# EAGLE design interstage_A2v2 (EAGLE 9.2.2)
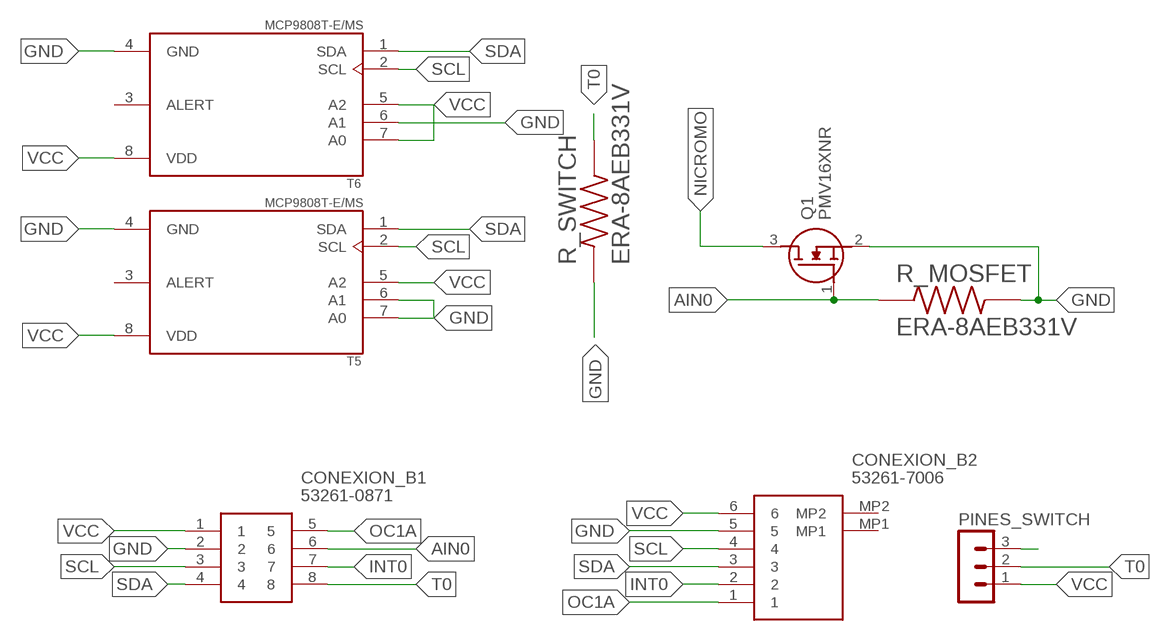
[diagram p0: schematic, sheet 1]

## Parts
CONEXION_B1  53261-0871  [53261-0871]
CONEXION_B2  53261-7006  [532617006]
PINES_SWITCH  MA03-1  [MA03-1]
Q1  PMV16XNR  [SOT95P230X110-3N]
R_MOSFET  ERA-8AEB331V  [RESC3216X70N]
R_SWITCH  ERA-8AEB331V  [RESC3216X70N]
T5  MCP9808T-E/MS  [SOP65P490X110-8N]
T6  MCP9808T-E/MS  [SOP65P490X110-8N]

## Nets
AIN0: CONEXION_B1.6 Q1.1(G) R_MOSFET.1
GND: CONEXION_B1.2 CONEXION_B2.5 Q1.2(S) R_MOSFET.2 R_SWITCH.1 T5.4(GND) T5.6(A1) T5.7(A0) T6.4(GND) T6.6(A1)
INT0: CONEXION_B1.7 CONEXION_B2.2
N$7: PINES_SWITCH.3
NICROMO: Q1.3(D)
OC1A: CONEXION_B1.5 CONEXION_B2.1
SCL: CONEXION_B1.3 CONEXION_B2.4 T5.2(SCL) T6.2(SCL)
SDA: CONEXION_B1.4 CONEXION_B2.3 T5.1(SDA) T6.1(SDA)
T0: CONEXION_B1.8 PINES_SWITCH.2 R_SWITCH.2
VCC: CONEXION_B1.1 CONEXION_B2.6 PINES_SWITCH.1 T5.5(A2) T5.8(VDD) T6.5(A2) T6.7(A0) T6.8(VDD)
Unconnected: CONEXION_B2.MP1 CONEXION_B2.MP2 T5.3(ALERT) T6.3(ALERT)

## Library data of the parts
CONEXION_B1 = SamacSys_Parts:53261-0871: Molex PICOBLADE Series, Series Number 53261, 1.25mm Pitch, 8 Way 1 Row Shrouded Right Angle PCB Header, Surface Mount Source: Datasheet; DESCRIPTION: Molex PICOBLADE Series, Series Number 53261, 1.25mm Pitch, 8 Way 1 Row Shrouded Right Angle PCB Header, Surface Mount; HEIGHT: mm; MANUFACTURER_NAME: Molex; MANUFACTURER_PART_NUMBER: 53261-0871; MOUSER_PART_NUMBER: 538-53261-0871; MOUSER_PRICE-STOCK: https://www.mouser.co.uk/ProductDetail/Molex/53261-0871?qs=%252B72YyncTwW%252BggfdCJ7Netw%3D%3D
CONEXION_B2 = SamacSys_Parts:53261-7006: 1.25mm Pitch, PicoBlade PCB Header, Single Row, Right-Angle, Surface Mount, Gold (Au) Plating, Friction Lock, Circuits, Tape and Reel Source: Datasheet; DESCRIPTION: 1.25mm Pitch, PicoBlade PCB Header, Single Row, Right-Angle, Surface Mount, Gold (Au) Plating, Friction Lock, Circuits, Tape and Reel; HEIGHT: 3.6mm; MANUFACTURER_NAME: Molex; MANUFACTURER_PART_NUMBER: 53261-7006; MOUSER_PART_NUMBER: 538-53261-7006; MOUSER_PRICE-STOCK: https://www.mouser.co.uk/ProductDetail/Molex/53261-7006?qs=0lSvoLzn4L%2FSBef0BTU2GA%3D%3D
PINES_SWITCH = con-lstb:MA03-1: PIN HEADER; OC_FARNELL: unknown; OC_NEWARK: unknown
Q1 = SamacSys_Parts:PMV16XNR: Nexperia PMV16XNR N-channel MOSFET, 8.6 A, 20 V PMV16XN, 3-Pin SOT-23 Source: Datasheet; DESCRIPTION: Nexperia PMV16XNR N-channel MOSFET, 8.6 A, 20 V PMV16XN, 3-Pin SOT-23; HEIGHT: 1.1mm; MANUFACTURER_NAME: Nexperia; MANUFACTURER_PART_NUMBER: PMV16XNR; MOUSER_PART_NUMBER: 771-PMV16XNR; MOUSER_PRICE-STOCK: https://www.mouser.com/Search/Refine.aspx?Keyword=771-PMV16XNR
R_MOSFET R_SWITCH = resistor_330_smd:ERA-8AEB331V; DESCRIPTION: 330 Ohms ±0.1% 0.25W, 1/4W Chip Resistor 1206 (3216 Metric) Automotive AEC-Q200 Thin Film; DIGI-KEY_PART_NUMBER: P330BCCT-ND; MF: Panasonic Electronic; MP: ERA-8AEB331V; PACKAGE: 3216 Panasonic Electronic Components
T5 T6 = sensorSPEL:MCP9808T-E/MS: Board Mount Temperature Sensors Silicon temp sensor with I2C interface; DESCRIPTION: Temperature Sensor Digital, Local -40°C ~ 125°C 10 b 8-MSOP; DIGI-KEY_PART_NUMBER: MCP9808T-E/MSCT-ND; MF: Microchip; MP: MCP9808T-E/MS; PACKAGE: MSOP-8 Microchip

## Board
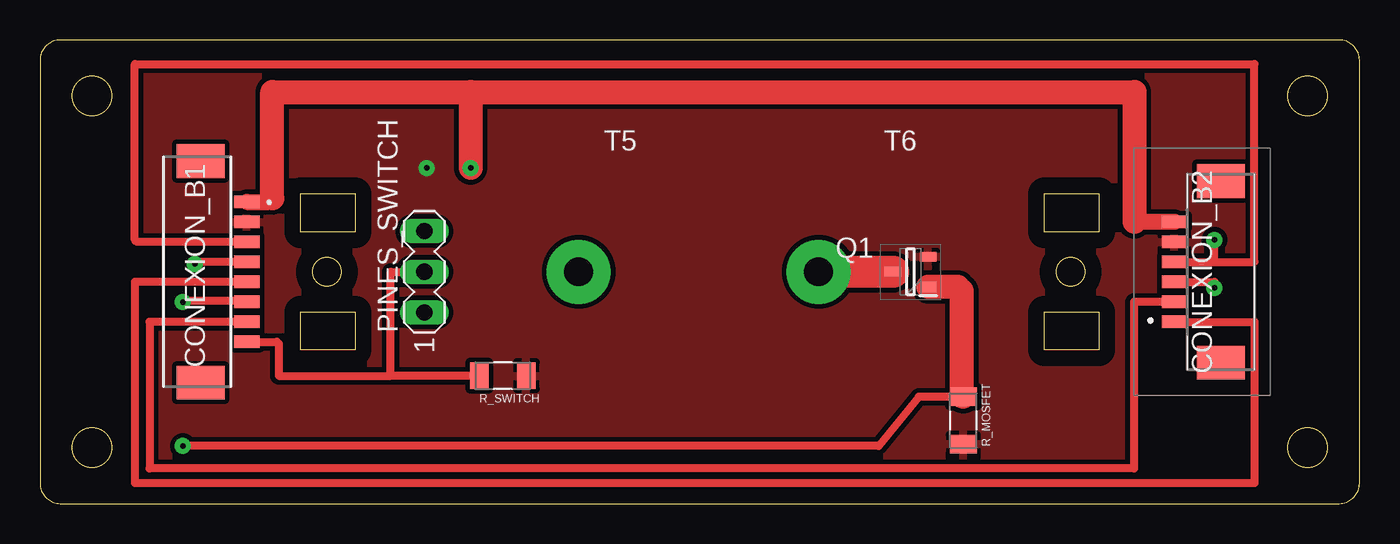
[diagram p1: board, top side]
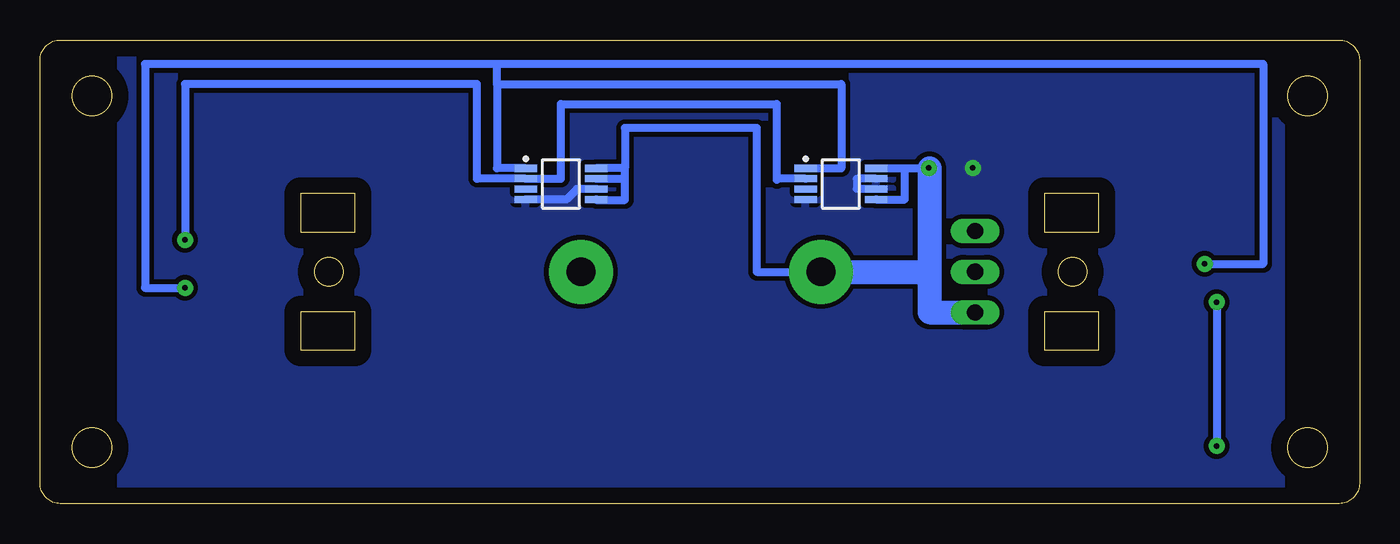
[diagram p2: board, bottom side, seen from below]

Size 82.5 x 29 mm. Coordinates in mm from the lower left corner, seen from the top.
Outline: 16.3,17 16.3,19.4 19.7,19.4 19.7,17 16.3,17
Outline: 62.8,9.6 62.8,12 66.2,12 66.2,9.6 62.8,9.6
Outline: 16.3,9.6 16.3,12 19.7,12 19.7,9.6 16.3,9.6
Outline: 62.8,17 62.8,19.4 66.2,19.4 66.2,17 62.8,17
Outline: 0,1.27 arc90 1.27,0 81.23,0 arc90 82.5,1.27 82.5,27.73 arc90 81.23,29 1.27,29 arc90 0,27.73 0,1.27
Outline: circle at 3.25,25.5 radius 1.25
Outline: circle at 79.25,3.5 radius 1.25
Outline: circle at 79.25,25.5 radius 1.25
Outline: circle at 3.25,3.5 radius 1.25
Outline: circle at 64.43,14.5 radius 0.9
Outline: circle at 17.93,14.5 radius 0.9
Copper layers (1*16): Top 0.035mm / dielectric 1.5mm / Bottom 0.035mm
Design rules "default *": minimum track width 6mil, minimum drill 0.35mm, track to track 0.3mm, track to pad 6mil, pad to pad 6mil, via to via 6mil, smd to smd 6mil, copper to edge 40mil, drill to drill 6mil, minimum pad ring 10mil, minimum via ring 8mil, stop-mask expansion 4mil, vias tented up to drill 0mil, thermal gap 10mil

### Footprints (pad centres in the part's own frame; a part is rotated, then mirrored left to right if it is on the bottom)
53261-0871 = smd 0.8 x 1.6: 1 -4.375,1.004; 2 -3.125,1.004; 3 -1.875,1.004; 4 -0.625,1.004; 5 0.625,1.004; 6 1.875,1.004; 7 3.125,1.004; 8 4.375,1.004 | smd 2.1 x 3: 9 6.925,-1.896; 10 -6.925,-1.896
532617006 = smd 0.8 x 1.6: 1 3.125,-2.5; 2 1.875,-2.5; 3 0.625,-2.5; 4 -0.625,-2.5; 5 -1.875,-2.5; 6 -3.125,-2.5 | smd 2.1 x 3: MP1 5.675,0.4; MP2 -5.675,0.4
MA03-1 = drill 1.016 long: 1 -2.54,0; 2 0,0; 3 2.54,0
SOT95P230X110-3N = smd 1.05 x 0.6: 1 -1.1,0.95; 2 -1.1,-0.95; 3 1.1,0
RESC3216X70N = smd 1.16 x 1.68: 1 -1.475,0; 2 1.475,0
SOP65P490X110-8N = smd 1.4 x 0.45: 1 -2.2,0.975; 2 -2.2,0.325; 3 -2.2,-0.325; 4 -2.2,-0.975; 5 2.2,-0.975; 6 2.2,-0.325; 7 2.2,0.325; 8 2.2,0.975

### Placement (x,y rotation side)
CONEXION_B1  11.93,14.5 270 top
CONEXION_B2  73.43,14.5 270 top
PINES_SWITCH  24.03,14.5 90 top
Q1  54.43,14.5 180 top
R_MOSFET  57.73,5.2 270 top
R_SWITCH  28.93,8 180 top
T5  32.43,20 0 bottom
T6  49.93,20 0 bottom

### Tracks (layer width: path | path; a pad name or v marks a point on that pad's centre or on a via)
AIN0  (via drill 0.35 pad 1)
  Top 0.5: 57.63,13.3 57.38,13.55 | v8.93,12.6 8.85,12.68 12.88,12.68 CONEXION_B1.6 | R_MOSFET.1 54.95,6.67 52.44,3.6 v8.93,3.6
  Top 1.5: R_MOSFET.1 57.63,6.7 57.63,13.3 | 57.38,13.55 Q1.1
  Bottom 0.5: v8.93,12.6 v8.93,3.6
GND  (via drill 0.35 pad 1)
  Bottom 0.5: T5.6 31.43,19.68 31.43,20.32 T5.7 | T6.6 48.93,19.68 49.58,19.02 T6.4
  other vias: 24.18,21
  pour Top (isolate 0.25): 4.93,28.3 4.93,0.5 77.43,0.5 77.43,28.3
  pour Bottom (isolate 0.25): 4.93,28.2 4.93,0.5 77.43,0.5 77.43,28.2
INT0
  Top 0.5: CONEXION_B1.7 6.85,11.38 6.85,2.19 68.41,2.19 68.41,12.62 CONEXION_B2.2
NICROMO  (via drill 1.8 pad 4)
  Top 2: Q1.3 v48.68,14.5
OC1A
  Top 0.5: CONEXION_B1.5 5.93,13.88 5.93,1.27 75.93,1.27 75.93,11.38 CONEXION_B2.1
SCL  (via drill 0.35 pad 1)
  Top 0.5: CONEXION_B1.3 6.05,16.38 5.93,16.5 5.93,27.5 75.93,27.5 75.93,15.12 73.43,15.12 | CONEXION_B2.4 73.43,15.12 | 73.43,15.12 v73.43,16.5
  Bottom 0.5: v73.43,16.5 73.43,26.25 55.18,26.25 55.18,20.32 T6.2 49.93,20.32 49.93,25 36.43,25 36.43,20.25 36.35,20.32 T5.2
SDA  (via drill 0.35 pad 1)
  Top 0.5: CONEXION_B1.4 9.8,15.12 v9.68,15 | CONEXION_B2.3 73.43,13.88 v73.43,13.5
  Bottom 0.5: T6.1 53.93,20.98 53.93,26.25 | 53.93,26.25 32.41,26.25 32.41,20.98 T5.1 | v9.68,15 6.03,15 6.03,27.5 53.93,27.5 | v73.43,13.5 75.93,13.5 75.93,27.5 53.93,27.5 | 53.93,26.25 53.93,27.5
T0
  Top 0.5: 21.93,8 21.93,14.5 PINES_SWITCH.2 | R_SWITCH.2 21.93,8 | CONEXION_B1.8 14.8,10.12 14.93,10 14.93,8 21.93,8
VCC  (via drill 0.35 pad 1, 1.8 pad 4)
  Top 0.5: 14.3,18.88 14.53,19.1
  Top 1: CONEXION_B1.1 14.3,18.88 | CONEXION_B2.6 68.43,17.62
  Top 1.5: 14.53,19.1 14.53,25.75 26.93,25.75 | 68.43,17.62 68.43,25.75 26.93,25.75 | 26.93,25.75 v26.93,21
  Bottom 0.5: T5.8 28.43,20.98 | 45.93,20.98 T6.8 | v26.93,21 26.41,21 26.39,20.98 26.89,20.98 28.43,20.98 | 45.93,20.98 45.93,23.5 37.68,23.5 37.68,14.5 v33.68,14.5 | T5.5 28.43,19.02 28.43,20.98 | T6.5 47.7,19 45.93,19 45.93,20.5 | 45.93,20.5 45.93,20.98 | T6.7 46.1,20.32 45.93,20.5
  Bottom 1.5: 26.89,20.98 26.89,14.5 | v33.68,14.5 26.89,14.5 | 26.89,14.5 26.89,11.96 PINES_SWITCH.1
